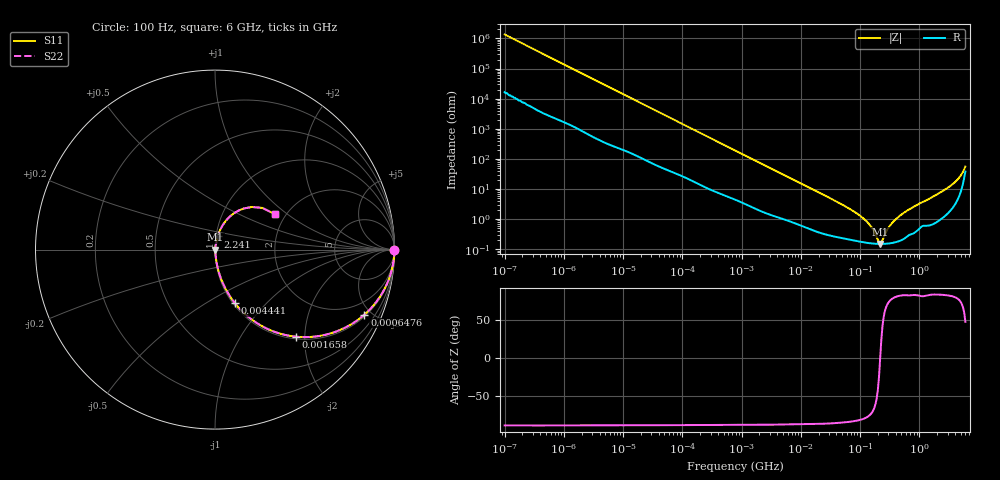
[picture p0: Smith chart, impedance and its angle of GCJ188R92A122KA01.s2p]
!Murata Part Number: GCJ188R92A122KA01
!These Parameters are Measured in Series Mode Connection
!Data Generated on Mar 13, 2026
!  o--ll--o
!Port1  Port2
!  o------o
!Operation Temp=25[degC], DC Bias Voltage=0[V]
!Freq. Start=100[Hz] Stop=6[GHz] 401[Steps]
# Hz S RI R 50
!Freq.(Hz) S11(Real) S11(Imag) S21(Real) S21(Imag) S12(Real) S12(Imag) S22(Real) S22(Imag)
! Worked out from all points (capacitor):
!   401 points, 100 Hz to 6 GHz, reference 50 ohm
!   read as one part in series: C = 1.17 nF near 109 Hz
!   lowest |Z| = 150 mohm at 218.4 MHz (marker M1)
!   series resonance near 218.9 MHz, so ESL is about 450 pH
!   S11 on the Smith chart (normalised r, x): 100 Hz: open; 647.6 kHz: 1.10, -4.55; 1.658 MHz: 1.05, -1.80; 4.441 MHz: 1.02, -0.68; 2.241 GHz: 1.02, +0.15; 6 GHz: 1.76, +0.82
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100  1 -7.35e-05  9e-07 7.35e-05  9e-07 7.35e-05  1 -7.35e-05
150  1 -0.00011  1.3e-06 0.00011  1.3e-06 0.00011  1 -0.00011
2008  1 -0.00144  1.98e-05 0.00144  1.98e-05 0.00144  1 -0.00144
40335  0.9988 -0.0282  0.00124 0.0282  0.00124 0.0282  0.9988 -0.0282
184852  0.9818 -0.1247  0.0182 0.1247  0.0182 0.1247  0.9818 -0.1247
647581  0.8324 -0.3624  0.1676 0.3624  0.1676 0.3624  0.8324 -0.3624
774597  0.7789 -0.4035  0.2211 0.4035  0.2211 0.4035  0.7789 -0.4035
1658239  0.4493 -0.485  0.5507 0.485  0.5507 0.485  0.4493 -0.485
4440638  0.1118 -0.2996  0.8882 0.2996  0.8882 0.2996  0.1118 -0.2996
1.555665e7  0.014 -0.0977  0.986 0.0977  0.986 0.0977  0.014 -0.0977
5.449875e7  0.00299 -0.0273  0.997 0.0273  0.997 0.0273  0.00299 -0.0273
1.020051e8  0.00191 -0.0124  0.9981 0.0124  0.9981 0.0124  0.00191 -0.0124
1.459435e8  0.00162 -0.0062  0.9984 0.0062  0.9984 0.0062  0.00162 -0.0062
1.996653e8  0.0015 -0.00138  0.9985 0.00138  0.9985 0.00138  0.0015 -0.00138
2.183701e8  0.00149 -3.87e-05  0.9985 3.87e-05  0.9985 3.87e-05  0.00149 -3.87e-05
2.388273e8  0.0015 0.00131  0.9985 -0.00131  0.9985 -0.00131  0.0015 0.00131
3.124326e8  0.00158 0.00547  0.9984 -0.00547  0.9984 -0.00547  0.00158 0.00547
4.087225e8  0.00183 0.01  0.9982 -0.01  0.9982 -0.01  0.00183 0.01
5.847788e8  0.00269 0.0174  0.9973 -0.0174  0.9973 -0.0174  0.00269 0.0174
2.240541e9  0.0148 0.0735  0.9852 -0.0735  0.9852 -0.0735  0.0148 0.0735
4.385646e9  0.0735 0.1751  0.9265 -0.1751  0.9265 -0.1751  0.0735 0.1751
6e9  0.3333 0.1978  0.6667 -0.1978  0.6667 -0.1978  0.3333 0.1978
